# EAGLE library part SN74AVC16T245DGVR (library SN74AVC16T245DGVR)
16-Bit Dual-Supply Bus Transceiver with Configurable Voltage-Level Shifting and 3-State Outputs Source: Datasheet
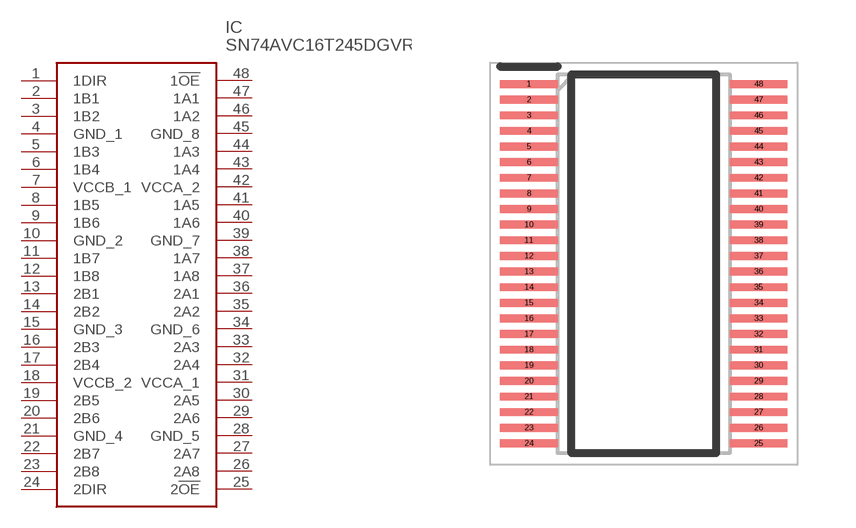
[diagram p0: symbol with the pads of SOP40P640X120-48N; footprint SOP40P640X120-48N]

Designator prefix IC

## SN74AVC16T245DGVR (Description: 16-Bit Dual-Supply Bus Transceiver with Configurable Voltage-Level Shifting and 3-State Outputs; Height: 1.2mm; Manufacturer_Name: Texas Instruments; Manufacturer_Part_Number: SN74AVC16T245DGVR; Mouser_Part_Number: 595-SN74AVC16T245DGV; Mouser_Price-Stock: https://www.mouser.co.uk/ProductDetail/Texas-Instruments/SN74AVC16T245DGVR?qs=PVVDbbWpW3LuulEdQVrkTg%3D%3D)  [SOP40P640X120-48N]
1  1DIR
2  1B1
3  1B2
4  GND_1
5  1B3
6  1B4
7  VCCB_1
8  1B5
9  1B6
10  GND_2
11  1B7
12  1B8
13  2B1
14  2B2
15  GND_3
16  2B3
17  2B4
18  VCCB_2
19  2B5
20  2B6
21  GND_4
22  2B7
23  2B8
24  2DIR
25  2!OE
26  2A8
27  2A7
28  GND_5
29  2A6
30  2A5
31  VCCA_1
32  2A4
33  2A3
34  GND_6
35  2A2
36  2A1
37  1A8
38  1A7
39  GND_7
40  1A6
41  1A5
42  VCCA_2
43  1A4
44  1A3
45  GND_8
46  1A2
47  1A1
48  1!OE

## Footprint SOP40P640X120-48N (pad centres in mm)
DGV (R-PDSO-G48)
smd 1.475 x 0.2: 1 -2.938,4.6; 2 -2.938,4.2; 3 -2.938,3.8; 4 -2.938,3.4; 5 -2.938,3; 6 -2.938,2.6; 7 -2.938,2.2; 8 -2.938,1.8; 9 -2.938,1.4; 10 -2.938,1; 11 -2.938,0.6; 12 -2.938,0.2; 13 -2.938,-0.2; 14 -2.938,-0.6; 15 -2.938,-1; 16 -2.938,-1.4; 17 -2.938,-1.8; 18 -2.938,-2.2; 19 -2.938,-2.6; 20 -2.938,-3; 21 -2.938,-3.4; 22 -2.938,-3.8; 23 -2.938,-4.2; 24 -2.938,-4.6; 25 2.938,-4.6; 26 2.938,-4.2; 27 2.938,-3.8; 28 2.938,-3.4; 29 2.938,-3; 30 2.938,-2.6; 31 2.938,-2.2; 32 2.938,-1.8; 33 2.938,-1.4; 34 2.938,-1; 35 2.938,-0.6; 36 2.938,-0.2; 37 2.938,0.2; 38 2.938,0.6; 39 2.938,1; 40 2.938,1.4; 41 2.938,1.8; 42 2.938,2.2; 43 2.938,2.6; 44 2.938,3; 45 2.938,3.4; 46 2.938,3.8; 47 2.938,4.2; 48 2.938,4.6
